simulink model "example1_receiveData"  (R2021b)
settings: Solver=FixedStepDiscrete  StartTime=0.0  StopTime=inf  FixedStep=0.2  RelTol=1e-3
undefined symbols (not defined in the file or in its folder): Big, Endian, Little
libraries: CANBusLib x3

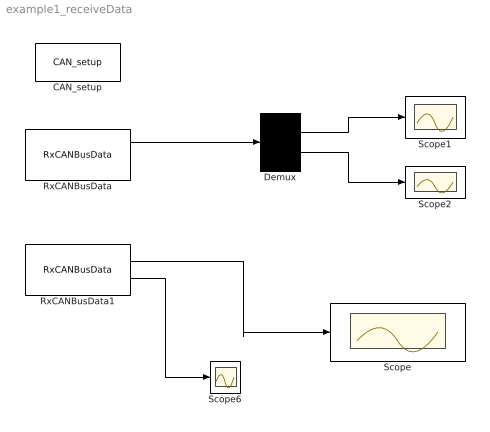
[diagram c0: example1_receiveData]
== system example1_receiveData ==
  CAN_setup : CANBusLib/CAN_setup  Priority=1  g1_cmbPortName="\"COM17\""  g2_cmbBaudRate=250000  g3_chkEcho=off  g59_chkTerminator=on  g4_cmbObjectID=0  g5_chkEnableSync=off  g10_chkRxWDEnable=off  g12_cmbRxWDLen=1  g13_cmbRxWDStartPos=1  g_60_cmbRxWDMode=0  g15_chkTxWDEnable=off  g17_cmbTxWDLen=1  g18_cmbTxWDStartPos=1  g_61_cmbTxWDMode=0  g20_ediF1=0  g21_chkExt4F1=off  g22_ediF2=0  g23_chkExt4F2=off  g24_ediF3=0  g25_chkExt4F3=off  g26_ediF4=0  g27_chkExt4F4=off  g28_ediF5=0  g29_chkExt4F5=off  g30_ediF6=0  g31_chkExt4F6=off  g32_ediF7=0  g33_chkExt4F7=off  g34_ediF8=0  g35_chkExt4F8=off  g36_ediM1=0  g37_ediF9=0  g38_chkExt4F9=on  g39_ediF10=0  g40_chkExt4F10=on  g41_ediF11=0  g42_chkExt4F11=on  g43_ediF12=0  g44_chkExt4F12=on  g45_ediM2=0  g46_ediF13=0  g47_chkExt4F13=off  g48_ediF14=0  g49_chkExt4F14=on  g50_ediF15=0  g51_chkExt4F15=on  g52_ediF16=0  g53_chkExt4F16=on  g54_ediM3=0  g62_autoFresh=on
  Demux : Demux  Outputs=2
  RxCANBusData : CANBusLib/RxCANBusData  g1_ObjectID=0  g2_CANID=888  g3_Extended=off  g4_Datatype="[ \"uint16\", \"uint8\"]"  g5_Endian=Little-Endian  g6_Longframe=off  g7_OutDataQTY=8  g8_FirstFrameNo=0
  RxCANBusData1 : CANBusLib/RxCANBusData  g1_ObjectID=0  g2_CANID=999  g3_Extended=on  g4_Datatype="\"int16\""  g5_Endian=Big-Endian  g6_Longframe=off  g7_OutDataQTY=5  g8_FirstFrameNo=0
  Scope{,1..2,6} (4 alike) : Scope
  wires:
  RxCANBusData1/1 -> Scope/1
  RxCANBusData1/2 -> Scope6/1
  RxCANBusData/1 -> Demux/1
  Demux/1 -> Scope1/1
  Demux/2 -> Scope2/1
